(* Logix 5000 AddOnInstructionDefinition export MCFG_Yaskawa; software revision 17.00; part 2 of 2 *)
(* tags used below, declared in another part *)
   Axis_OUT : AB:ETHERNET_MODULE_DINT_256Bytes:O:0;
   Axis : Yaskawa_EIP_Servo;
(* MCFG_Yaskawa, continued *)

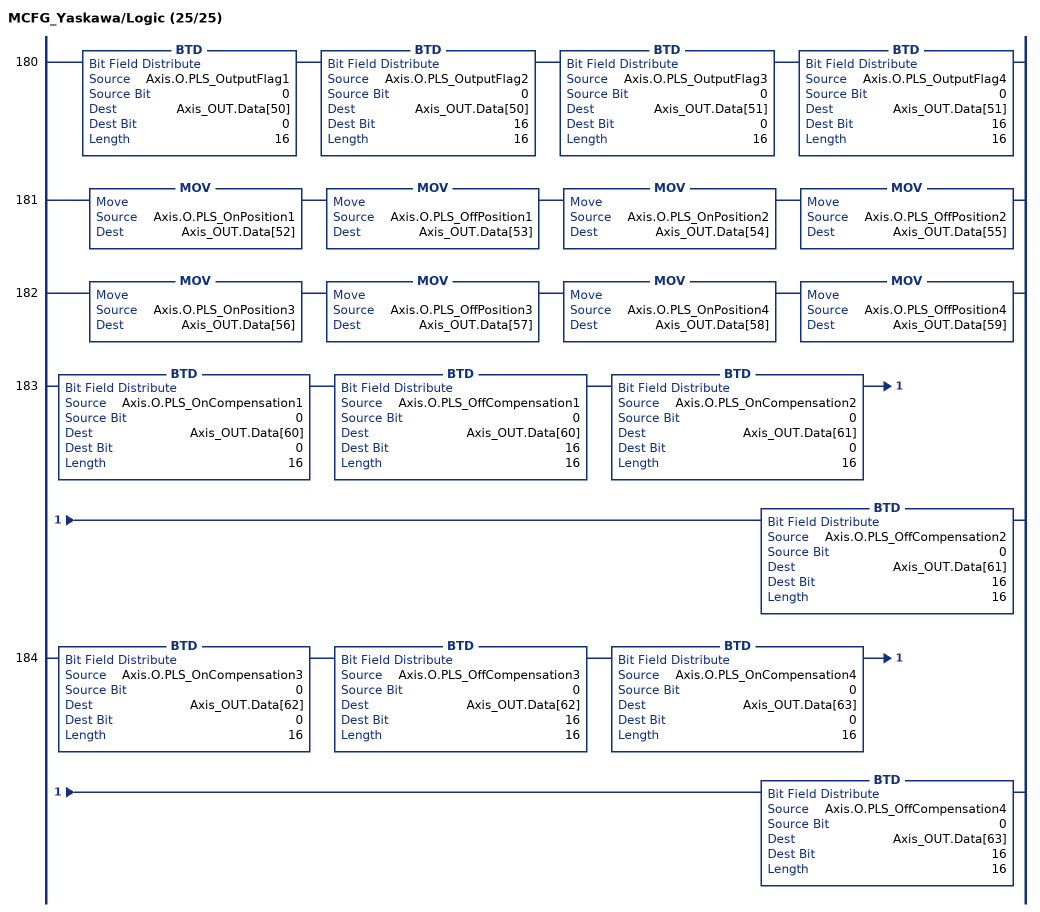
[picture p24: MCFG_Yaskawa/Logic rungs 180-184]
   180: BTD(Axis.O.PLS_OutputFlag1,0,Axis_OUT.Data[50],0,16)BTD(Axis.O.PLS_OutputFlag2,0,Axis_OUT.Data[50],16,16)BTD(Axis.O.PLS_OutputFlag3,0,Axis_OUT.Data[51],0,16)BTD(Axis.O.PLS_OutputFlag4,0,Axis_OUT.Data[51],16,16);
   181: MOV(Axis.O.PLS_OnPosition1,Axis_OUT.Data[52])MOV(Axis.O.PLS_OffPosition1,Axis_OUT.Data[53])MOV(Axis.O.PLS_OnPosition2,Axis_OUT.Data[54])MOV(Axis.O.PLS_OffPosition2,Axis_OUT.Data[55]);
   182: MOV(Axis.O.PLS_OnPosition3,Axis_OUT.Data[56])MOV(Axis.O.PLS_OffPosition3,Axis_OUT.Data[57])MOV(Axis.O.PLS_OnPosition4,Axis_OUT.Data[58])MOV(Axis.O.PLS_OffPosition4,Axis_OUT.Data[59]);
   183: BTD(Axis.O.PLS_OnCompensation1,0,Axis_OUT.Data[60],0,16)BTD(Axis.O.PLS_OffCompensation1,0,Axis_OUT.Data[60],16,16)BTD(Axis.O.PLS_OnCompensation2,0,Axis_OUT.Data[61],0,16)BTD(Axis.O.PLS_OffCompensation2,0,Axis_OUT.Data[61],16,16);
   184: BTD(Axis.O.PLS_OnCompensation3,0,Axis_OUT.Data[62],0,16)BTD(Axis.O.PLS_OffCompensation3,0,Axis_OUT.Data[62],16,16)BTD(Axis.O.PLS_OnCompensation4,0,Axis_OUT.Data[63],0,16)BTD(Axis.O.PLS_OffCompensation4,0,Axis_OUT.Data[63],16,16);
END_ROUTINE

ROUTINE Prescan   (* ladder *)
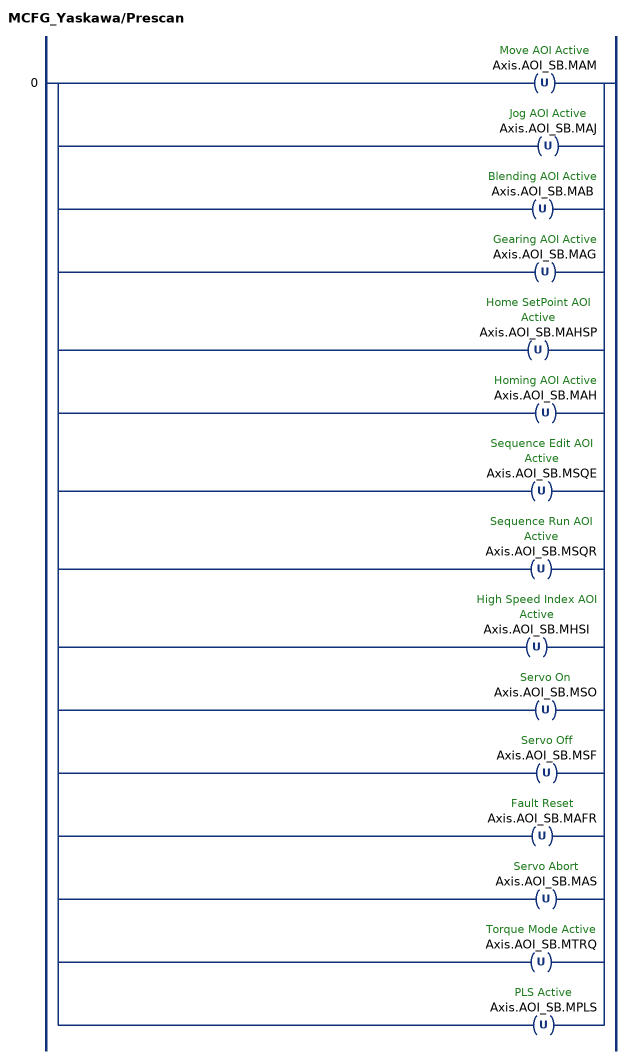
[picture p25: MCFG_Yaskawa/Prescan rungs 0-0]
   0: [OTU(Axis.AOI_SB.MAM) ,OTU(Axis.AOI_SB.MAJ) ,OTU(Axis.AOI_SB.MAB) ,OTU(Axis.AOI_SB.MAG) ,OTU(Axis.AOI_SB.MAHSP) ,OTU(Axis.AOI_SB.MAH) ,OTU(Axis.AOI_SB.MSQE) ,OTU(Axis.AOI_SB.MSQR) ,OTU(Axis.AOI_SB.MHSI) ,OTU(Axis.AOI_SB.MSO) ,OTU(Axis.AOI_SB.MSF) ,OTU(Axis.AOI_SB.MAFR) ,OTU(Axis.AOI_SB.MAS) ,OTU(Axis.AOI_SB.MTRQ) ,OTU(Axis.AOI_SB.MPLS) ];
END_ROUTINE
END_ADD_ON_INSTRUCTION
